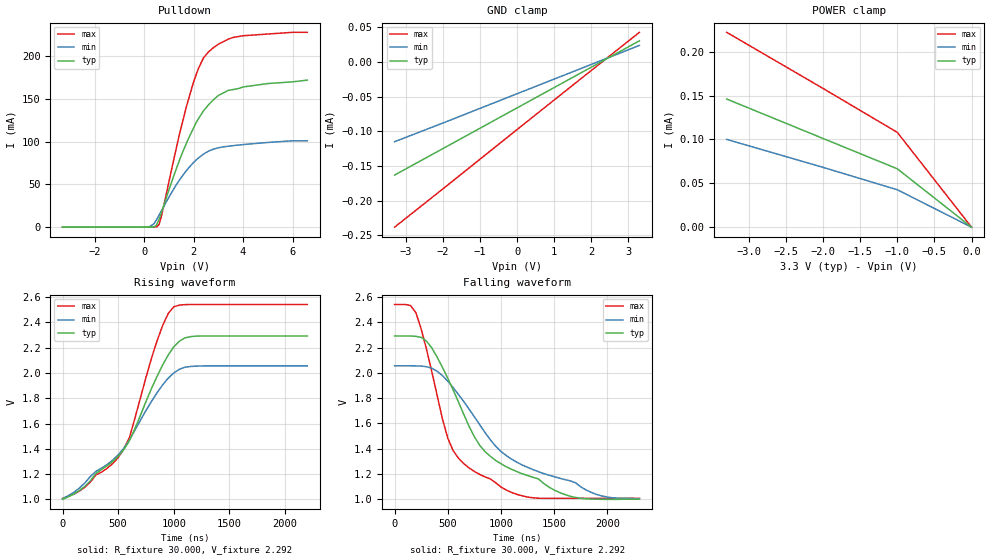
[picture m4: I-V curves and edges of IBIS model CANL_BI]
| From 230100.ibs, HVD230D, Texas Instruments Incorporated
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[Model]   CANL_BI
Model_type   I/O_open_drain
| Signals   CANL
Vinh = 0.9V
Vinl = 0.5V
Rref = 30   |Note: 60 Ohm differential load;
Vref = 2.3   |tr,tf measured in single ended configuration
| variable   typ   min   max
C_comp   30.0pF   24.0pF   36.0pF
|   typ   min   max
[Temperature Range]   25.0   -40   85
[Voltage range]   3.3V   3.0V   3.6V
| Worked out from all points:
|   slope of the pulldown table from 0 to 0.495 V, typ, clamps not added: 228 ohm
|   rising waveform, R_fixture 30.000, V_fixture 2.292: 20-80 % time 495ns typ, 559ns min, 359ns max; typ from 1 V to 2.29 V
|   falling waveform, R_fixture 30.000, V_fixture 2.292: 20-80 % time 590ns typ, 775ns min, 328ns max; typ from 2.29 V to 1 V
[Pulldown]
|   Voltage   I(typ)   I(min)   I(max)
-3.3V     -165uA     -149uA     -186uA
200mV     -62uA      33.4uA     -75uA
500mV     2.21mA     8.47mA     -6.56uA
600mV     8.65mA     13.7mA     2.61mA
700mV     16.9mA     19mA       12.7mA
1.4V      75.9mA     53.7mA     105mA
1.7V      97.5mA     65.7mA     140mA
2V        116mA      75.6mA     170mA
2.4V      136mA      85.4mA     198mA
3V        154mA      92.8mA     214mA
3.4V      160mA      94.6mA     220mA
6.6V      172mA      101mA      228mA
[Power_clamp]
| Note that the[POWER_clamp]voltage table is referenced to Vcc
| and is calculated using Vtable=Vcc - Vmeasured.
|   Voltage   I(typ)   I(min)   I(max)
-3.3V     146uA      100uA      222uA
-2V       101uA      68.1uA     158uA
-1V       66.5uA     42.6uA     108uA
0V        0A         0A         0A
[GND_clamp]
|   Voltage   I(typ)   I(min)   I(max)
-3.3V     -163uA     -115uA     -238uA
-2V       -125uA     -88.2uA    -183uA
0V        -66.4uA    -46uA      -97.6uA
1.5V      -22.5uA    -14.4uA    -33.8uA
3.3V      30.2uA     23.6uA     42.4uA
[Ramp]
|   typ   min   max
dV/dt_r   0.775/496ns   0.636/557ns   0.920/358ns
dV/dt_f   0.714/594ns   0.636/775ns   0.920/328ns
R_load = 30ohm  | Note: The measurement is single-ended with 30ohm
|   to Vfixture.
[Rising Waveform]
R_fixture = 30.000
V_fixture = 2.292
V_fixture_min = 2.055
V_fixture_max = 2.541
C_fixture = 0.000
L_fixture = 0.000
|  time   V(typ)   V(min)   V(max)
0s        1.001V     1.006V     1.008V
200ns     1.103V     1.13V      1.096V
450ns     1.3V       1.31V      1.283V
550ns     1.393V     1.404V     1.399V
600ns     1.462V     1.468V     1.486V
850ns     1.974V     1.844V     2.255V
950ns     2.142V     1.959V     2.47V
1us       2.207V     2V         2.523V
1.2us     2.291V     2.054V     2.541V
2.2us     2.292V     2.056V     2.541V
[Falling Waveform]
R_fixture = 30.000
V_fixture = 2.292
V_fixture_min = 2.055
V_fixture_max = 2.541
C_fixture = 0.000
L_fixture = 0.000
|  time   V(typ)   V(min)   V(max)
0s        2.292V     2.056V     2.541V
200ns     2.289V     2.055V     2.477V
350ns     2.197V     2.037V     2.008V
500ns     1.957V     1.934V     1.483V
700ns     1.577V     1.713V     1.248V
850ns     1.377V     1.528V     1.177V
1.15us    1.219V     1.293V     1.039V
1.65us    1.024V     1.146V     1.008V
1.95us    1V         1.026V     1.008V
2.3us     1.001V     1.006V     1.008V
